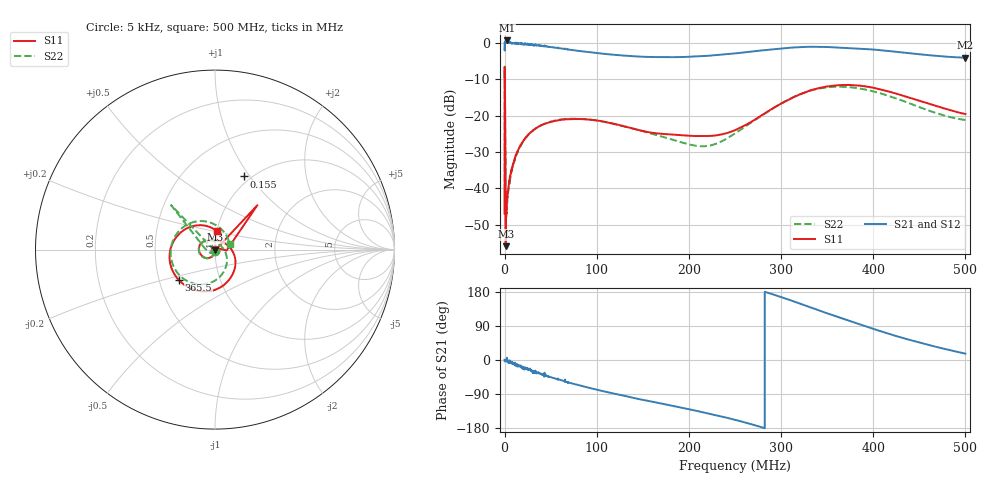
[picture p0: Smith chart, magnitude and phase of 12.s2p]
#  HZ  S  MA  R  50.00
! Rohde & Schwarz Vector Network Analyzer
! Rohde-Schwarz,ZNL6-2Port,1323001206101378,1.50.1.34-21.10.1.104
! Created: UTC 10/21/2024, 2:39:58 AM
! freq[Hz]  mag:S11  ang:S11  mag:S21  ang:S21  mag:S12  ang:S12  mag:S22  ang:S22
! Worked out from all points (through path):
!   10001 points, 5 kHz to 500 MHz, reference 50 ohm
!   highest |S21| = 0.65 dB at 2.505 MHz (marker M1); lowest = -4.1 dB at 500 MHz (marker M2)
!   group delay of S21, straight-line fit = 1.87 ns
!   lowest |S11| = -55.8 dB at 1.155 MHz (marker M3), VSWR 1.00, Z = 50.1 - j0.12 ohm
!   |S11| at or under -10 dB: start of sweep to 50.87 kHz; 337.1 kHz to end of sweep
!   |S22| runs from -47.8 to -6.5 dB; largest |S21 - S12| = 0.33
!   S11 on the Smith chart (normalised r, x): 5 kHz: 1.00, -0.01; 155 kHz: 0.93, +0.93; 365.5 MHz: 0.63, -0.23; 500 MHz: 1.00, +0.21
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5000  0.004471 -89.0  0.9998 0.7  0.9992 0.4  0.006526 -100.3
154998.5  0.4375 68.7  0.8085 -2.5  0.7852 -1.2  0.4426 114.2
1154988  0.001615 -47.8  1 -1.1  0.999 -1.0  0.008554 -60.3
2504975  0.007462 -80.1  1.078 5.8  0.8921 -10.2  0.005505 -76.2
3104969  0.007726 -84.6  1 -5.1  0.9909 -1.6  0.007088 -78.5
3654964  0.00935 -87.3  1.018 -2.3  0.9749 -5.5  0.008441 -81.3
7304927  0.01768 -96.7  0.9936 -5.7  0.9899 -8.6  0.01669 -92.1
1.310487e7  0.03057 -105.4  0.9864 -12.8  0.9841 -12.4  0.0294 -102.6
2.96047e7  0.06121 -129.1  0.9406 -28.4  0.9518 -26.8  0.06067 -127.7
5.545445e7  0.08497 -163.4  0.8566 -49.4  0.8602 -48.0  0.08609 -160.8
8.335417e7  0.08964 168.5  0.7663 -68.3  0.7692 -67.3  0.09012 171.1
1.234038e8  0.07483 141.5  0.6776 -91.1  0.6801 -90.5  0.07482 140.6
1.667033e8  0.05695 114.4  0.6367 -113.2  0.6392 -112.4  0.05335 108.4
2.161028e8  0.05235 79.1  0.658 -138.3  0.6589 -137.2  0.038 47.2
2.500025e8  0.06321 36.0  0.7158 -157.8  0.7159 -156.3  0.05701 -10.6
2.97002e8  0.1393 -35.2  0.8309 168.5  0.8333 170.7  0.1393 -72.0
3.333517e8  0.2255 -90.6  0.8832 137.9  0.8884 140.7  0.2234 -122.2
3.655013e8  0.2634 -140.2  0.8586 110.2  0.8642 113.0  0.2495 -168.8
3.903011e8  0.2538 -174.5  0.8255 90.1  0.8302 92.4  0.2297 156.3
4.167008e8  0.2146 154.2  0.7727 69.3  0.7724 71.3  0.1872 122.9
4.552504e8  0.1533 117.8  0.6867 42.8  0.6884 44.2  0.1238 77.1
5e8  0.1053 82.8  0.625 16.7  0.6242 17.7  0.08714 20.9
